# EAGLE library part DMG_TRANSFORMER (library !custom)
Strange little transformer used in the DMG DC power conversion board. Symbol is based largely off the pre-existing schematic at Gbdev. Part is about as accurate as it can be without the original spec.
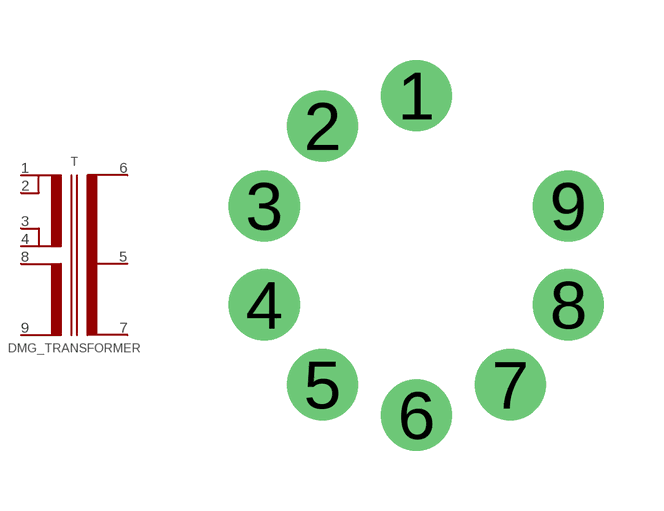
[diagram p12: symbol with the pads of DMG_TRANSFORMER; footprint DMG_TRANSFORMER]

Designator prefix T

## DMG_TRANSFORMER  [DMG_TRANSFORMER]
1  1  pas
2  2  pas
3  3  pas
4  4  pas
5  5  pas
6  6  pas
7  7  pas
8  8  pas
9  9  pas

## Footprint DMG_TRANSFORMER (pad centres in mm)
drill 1.016 pad 1.778: 1 0,4; 2 -2.351,3.236; 3 -3.804,1.236; 4 -3.804,-1.236; 5 -2.351,-3.236; 6 0,-4; 7 2.351,-3.236; 8 3.804,-1.236; 9 3.804,1.236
